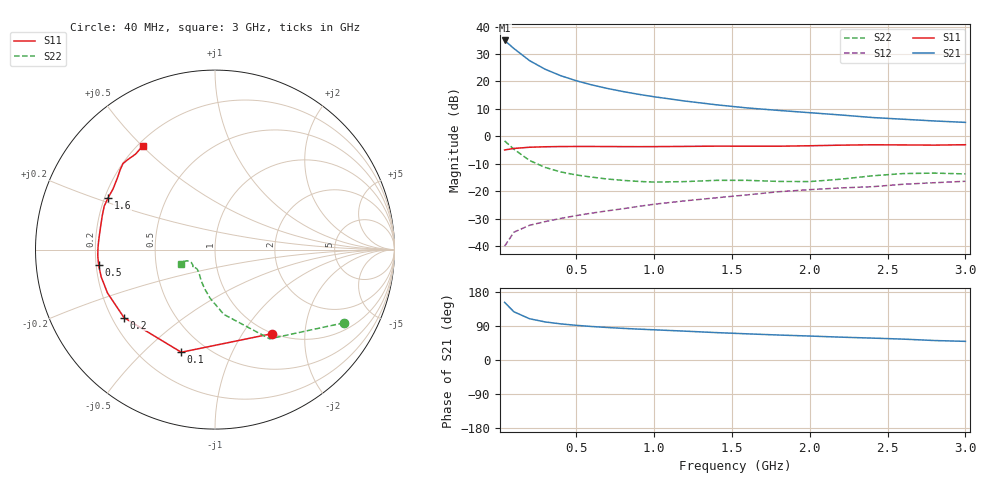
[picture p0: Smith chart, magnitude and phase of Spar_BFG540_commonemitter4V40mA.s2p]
! Filename:  BFG540E.S2P  Version:  3.0
! NXP part #: BFG540  Date: Feb 1992
! Bias condition: Vce=4V, Ic=40mA
! IN LINE PINNING: same data as with cross emitter pinning.
#  MHz  S  MA  R  50
! Freq  S11  S21  S12  S22  !GUM [dB]
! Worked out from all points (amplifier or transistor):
!   21 points, 40 MHz to 3 GHz, reference 50 ohm
!   highest |S21| = 34.9 dB at 40 MHz (marker M1)
!   |S21| within 3 dB of that: start of sweep to 101.2 MHz
!   unconditionally stable (mu >= 1): 684.1 MHz to end of sweep
!   at 300 MHz: K = 0.68, MSG = 27.8 dB, |S12| = -31.1 dB
!   at 1 GHz: K = 1.11, MAG = 17.6 dB, |S12| = -24.7 dB
!   at 3 GHz: K = 1.14, MAG = 8.4 dB, |S12| = -16.4 dB
!   lowest NFmin = 1.90 dB at 900 MHz
!   S11 on the Smith chart (normalised r, x): 40 MHz: 0.99, -1.36; 100 MHz: 0.37, -0.66; 200 MHz: 0.25, -0.31; 500 MHz: 0.21, -0.06; 1.6 GHz: 0.21, +0.22; 3 GHz: 0.22, +0.50
40  0.565 -56.1  55.76 152.1  0.01 68.6  0.826 -29.6
100  0.602 -108.2  39.71 127.2  0.018 51.9  0.583 -58.5
200  0.633 -143.2  23.95 108.9  0.024 46.1  0.364 -82.3
300  0.646 -158.1  16.69 100.5  0.028 47.3  0.272 -95.8
400  0.652 -166.5  12.74 95.3  0.032 51.0  0.225 -104.9
500  0.654 -172.3  10.3 91.5  0.036 53.9  0.198 -111.5
600  0.654 -177.0  8.651 88.4  0.04 56.7  0.181 -116.4
700  0.652 179.1  7.453 85.8  0.044 59.0  0.167 -120.7
800  0.65 175.6  6.547 83.5  0.048 60.9  0.158 -124.6
900  0.649 172.2  5.831 81.5  0.053 62.5  0.151 -128.8
1000  0.65 168.8  5.261 79.7  0.058 63.9  0.147 -132.8
1200  0.656 163.2  4.39 76.1  0.067 65.5  0.15 -139.0
1400  0.663 158.6  3.756 72.3  0.076 65.8  0.158 -141.1
1600  0.662 154.2  3.288 69.0  0.086 67.5  0.158 -141.5
1800  0.661 149.2  2.967 65.9  0.098 66.9  0.151 -144.0
2000  0.674 143.9  2.696 63.2  0.107 67.5  0.15 -151.1
2200  0.691 139.8  2.449 60.3  0.115 67.2  0.166 -158.0
2400  0.702 136.9  2.205 57.8  0.121 67.7  0.191 -159.6
2600  0.698 134.0  2.049 55.1  0.134 66.5  0.21 -157.1
2800  0.692 129.8  1.907 51.4  0.143 64.0  0.214 -154.6
3000  0.704 124.8  1.796 49.2  0.152 64.5  0.207 -156.5
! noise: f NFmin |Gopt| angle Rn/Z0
900  1.9  0.351  179  0.11
2000  2.6  0.543  -150  0.17
